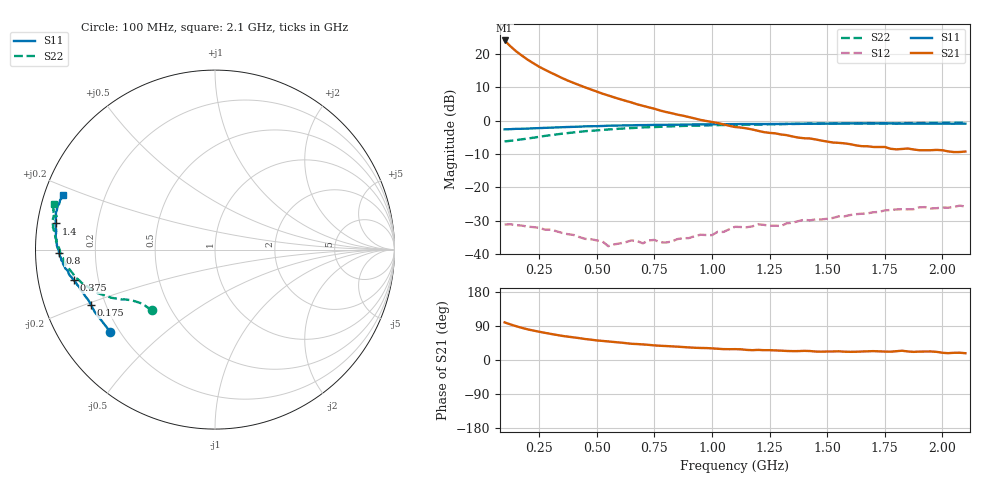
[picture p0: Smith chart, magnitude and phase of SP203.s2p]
!  POLYFET RF DEVICES
!  S PARAMETERS FOR
!  SP203
!  VDS=28, IDQ=600MA
! Date: Thu Sep 24 14:56:05 1998
! S2A 3Die, AP pkg, Vds=28Vdc, Idq=600ma, Vgsth=3.35Vdc,
# MHZ  S  MA  R  50.0000
! SCATTERING PARAMETERS :
! Freq=MHz Mag[s11] Ang[s11] Mag[s21] Ang[s21] Mag[s12] Ang[s12] Mag[s22] Ang[s22]
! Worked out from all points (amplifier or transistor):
!   81 points, 100 MHz to 2.1 GHz, reference 50 ohm
!   highest |S21| = 24.1 dB at 100 MHz (marker M1)
!   |S21| within 3 dB of that: start of sweep to 145.9 MHz
!   unconditionally stable (mu >= 1): 420.8 MHz to end of sweep
!   at 425 MHz: K = 1.02, MAG = 21.9 dB, |S12| = -35.0 dB
!   at 1.1 GHz: K = 1.50, MAG = 10.8 dB, |S12| = -31.9 dB
!   at 2.1 GHz: K = 1.30, MAG = 4.9 dB, |S12| = -25.8 dB
!   S11 on the Smith chart (normalised r, x): 100 MHz: 0.17, -0.34; 175 MHz: 0.15, -0.21; 375 MHz: 0.11, -0.11; 800 MHz: 0.07, -0.01; 1.4 GHz: 0.05, +0.08; 2.1 GHz: 0.05, +0.17
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100  0.7427 -141.7  16.04 99.3  0.02759 10.1  0.4888 -136.2
125  0.7458 -148.0  13.13 94.0  0.02784 7.4  0.4988 -141.1
150  0.7548 -152.5  11.03 89.2  0.02701 3.7  0.5111 -144.3
175  0.7563 -155.8  9.5 84.8  0.02658 1.0  0.5252 -146.4
200  0.7601 -158.4  8.254 80.9  0.02565 -0.0  0.5393 -148.2
225  0.7692 -160.5  7.286 77.7  0.02522 -0.5  0.5556 -149.7
250  0.7736 -162.0  6.462 74.6  0.02465 -3.2  0.5728 -151.0
300  0.7858 -164.8  5.281 68.9  0.02312 -2.8  0.6058 -153.1
350  0.7982 -167.0  4.359 63.6  0.0206 -4.9  0.6377 -155.1
375  0.8046 -167.7  3.996 61.7  0.01973 -0.3  0.6522 -156.5
450  0.8232 -170.0  3.162 55.3  0.0168 4.5  0.6959 -159.5
500  0.8267 -171.6  2.739 51.7  0.01594 9.9  0.7154 -161.6
575  0.8426 -173.5  2.243 47.5  0.01387 20.8  0.7476 -164.4
650  0.8506 -175.6  1.881 42.8  0.01591 30.0  0.7743 -167.1
775  0.8656 -178.0  1.422 37.5  0.01493 45.9  0.8087 -171.1
800  0.867 -178.7  1.352 36.9  0.0148 47.2  0.8154 -172.0
1100  0.8891 175.6  0.8047 28.6  0.02549 72.9  0.8652 -179.9
1300  0.8947 172.4  0.6209 24.7  0.02623 75.5  0.8872 176.3
1400  0.8988 170.7  0.5451 24.1  0.03256 80.1  0.8985 174.3
1450  0.9003 170.1  0.5232 22.3  0.03303 83.5  0.9019 173.4
1775  0.9092 164.5  0.379 21.9  0.04562 83.8  0.9185 168.2
2100  0.9016 160.4  0.3443 18.0  0.05149 80.4  0.9297 164.2
